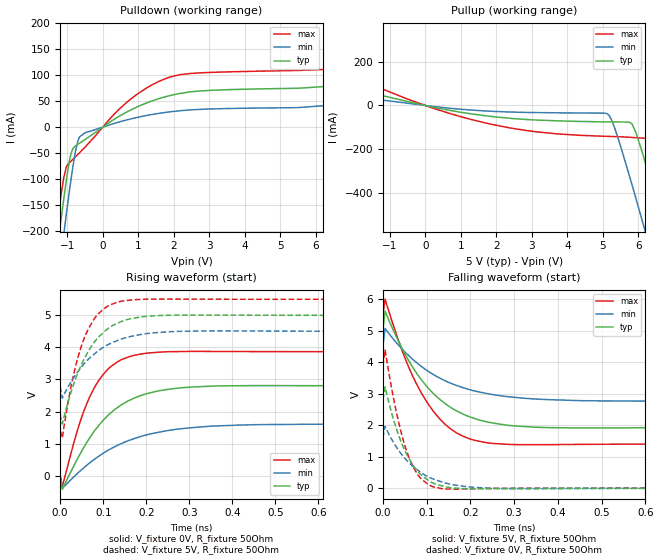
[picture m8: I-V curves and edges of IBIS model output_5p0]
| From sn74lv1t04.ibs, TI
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|   output_5p0 Model
[Model]   output_5p0
Model_type   Output
Polarity   Inverting
Vmeas = 2.5
Vref = 0
Cref = 30pF
Rref = 100
|   typ   min   max
|   (nom PVT)   (fast PVT)   (slow PVT)
C_comp   2.130e-12   2.046e-12   2.155e-12
| Where nom  PVT is Nominal Process, 5V, 40C
|   Fast PVT is Strong Process,  5.5V, -40C
|   Slow PVT is Weak Process,   4.5V, 140C
[Voltage Range]   5   4.5   5.5
|Junction Temperature
[Temperature Range]   40   140   -40
[Pullup Reference]   5   4.5   5.5
[Pulldown Reference]   0   0   0
[Power Clamp Reference]   5   4.5   5.5
[GND Clamp Reference]   0   0   0
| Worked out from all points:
|   slope of the pulldown table from 0 to 0.75 V, typ, clamps not added: 23.6 ohm
|   slope of the pullup table from 0 to 0.75 V, typ, clamps not added: 31.2 ohm
|   falling waveform, V_fixture 5V, R_fixture 50Ohm: 20-80 % time 112ps typ, 136ps min, 92.9ps max; typ from 5 V to 1.93 V
|   rising waveform, V_fixture 0V, R_fixture 50Ohm: 20-80 % time 104ps typ, 140ps min, 69.9ps max; typ from 0 V to 2.8 V
|   rising waveform, V_fixture 5V, R_fixture 50Ohm: 20-80 % time 70.5ps typ, 87.9ps min, 52.4ps max; typ from 1.93 V to 5 V
|   falling waveform, V_fixture 0V, R_fixture 50Ohm: 20-80 % time 55ps typ, 78ps min, 45.2ps max; typ from 2.8 V to 0 V
[Pulldown]
|   Voltage   I(typ)   I(min)   I(max)
-5V       -2.428A    -2.493A    -2.381A
-1.573V   -402.3mA   -473mA     -351mA
-1.216V   -201.1mA   -271mA     -152.2mA
-1.101V   -139.7mA   -207.8mA   -97.86mA
-1.024V   -101.5mA   -166.7mA   -76.37mA
-885mV    -49.18mA   -96.81mA   -65.02mA
-761mV    -35.83mA   -44.2mA    -56.81mA
-657.5mV  -31.1mA    -18.96mA   -49.77mA
692.5mV   29.77mA    14.17mA    48.77mA
1.804V    59.33mA    28.77mA    94.53mA
6.45V     79.41mA    42.64mA    112.1mA
10V       154mA      89.04mA    216.4mA
[Pullup]
|   Voltage   I(typ)   I(min)   I(max)
-5V       197.7mA    96.51mA    357.2mA
-2.845V   107.2mA    57.4mA     181.5mA
700mV     -22.65mA   -12.82mA   -37.2mA
2.911V    -64.77mA   -31.87mA   -116mA
5.082V    -74.99mA   -35.48mA   -141.1mA
5.292V    -75.21mA   -84.78mA   -142.1mA
5.825V    -85.33mA   -364.8mA   -146.2mA
6.12V     -219.3mA   -533.2mA   -149.2mA
6.446V    -401.4mA   -721.8mA   -152.5mA
6.731V    -566.4mA   -888.9mA   -290.8mA
7.226V    -856mA     -1.151A    -573.2mA
10V       -2.424A    -2.787A    -2.079A
[Ramp]
R_load = 50
|   typ   min   max
dV/dt_r   1.6784/1.04165e-10   0.955256/1.39794e-10   2.3196/6.9889e-11
dV/dt_f   1.84348/1.1157e-10   1.03365/1.36462e-10   2.46005/9.29136e-11
[Falling Waveform]
V_fixture = 5V
V_fixture_min = 4.5V
V_fixture_max = 5.5V
R_fixture = 50Ohm
|   Time   V(typ)   V(min)   V(max)
0s        5V         4.5V       5.5V
5ps       5.618V     5.065V     5.997V
35ps      4.68V      4.549V     4.711V
60ps      4.024V     4.191V     3.809V
90ps      3.404V     3.841V     2.973V
120ps     2.941V     3.568V     2.361V
170ps     2.443V     3.251V     1.743V
240ps     2.097V     2.997V     1.44V
465ps     1.911V     2.774V     1.392V
1.985ns   1.928V     2.778V     1.4V
[Rising Waveform]
V_fixture = 0V
V_fixture_min = 0V
V_fixture_max = 0V
R_fixture = 50Ohm
|   Time   V(typ)   V(min)   V(max)
0s        538pV      3.382nV    1.364nV
5ps       -420mV     -398.5mV   -335mV
50ps      765.6mV    189.8mV    1.825V
70ps      1.208V     413.2mV    2.493V
90ps      1.571V     610.5mV    2.975V
135ps     2.14V      957.8mV    3.563V
200ps     2.552V     1.27V      3.818V
295ps     2.756V     1.482V     3.874V
460ps     2.809V     1.592V     3.869V
2.01ns    2.797V     1.591V     3.866V
[Rising Waveform]
V_fixture = 5V
V_fixture_min = 4.5V
V_fixture_max = 5.5V
R_fixture = 50Ohm
|   Time   V(typ)   V(min)   V(max)
0s        1.928V     2.777V     1.4V
5ps       1.616V     2.419V     1.179V
20ps      2.373V     2.805V     2.416V
30ps      2.797V     3.028V     3.081V
45ps      3.33V      3.314V     3.855V
60ps      3.744V     3.554V     4.417V
90ps      4.331V     3.908V     5.066V
135ps     4.763V     4.225V     5.415V
270ps     5.006V     4.498V     5.505V
1.015ns   5V         4.499V     5.5V
[Falling Waveform]
V_fixture = 0V
V_fixture_min = 0V
V_fixture_max = 0V
R_fixture = 50Ohm
|   Time   V(typ)   V(min)   V(max)
0s        2.799V     1.592V     3.872V
5ps       3.216V     1.963V     4.383V
20ps      2.388V     1.553V     3.17V
35ps      1.72V      1.22V      2.158V
60ps      939.2mV    802.4mV    967.2mV
85ps      455.7mV    520.7mV    336.5mV
115ps     162.1mV    292.6mV    44.81mV
160ps     8.748mV    113.5mV    -27.14mV
265ps     -11.96mV   -5.667mV   -3.19mV
990ps     -10.12uV   618.3uV    -25.24uV
